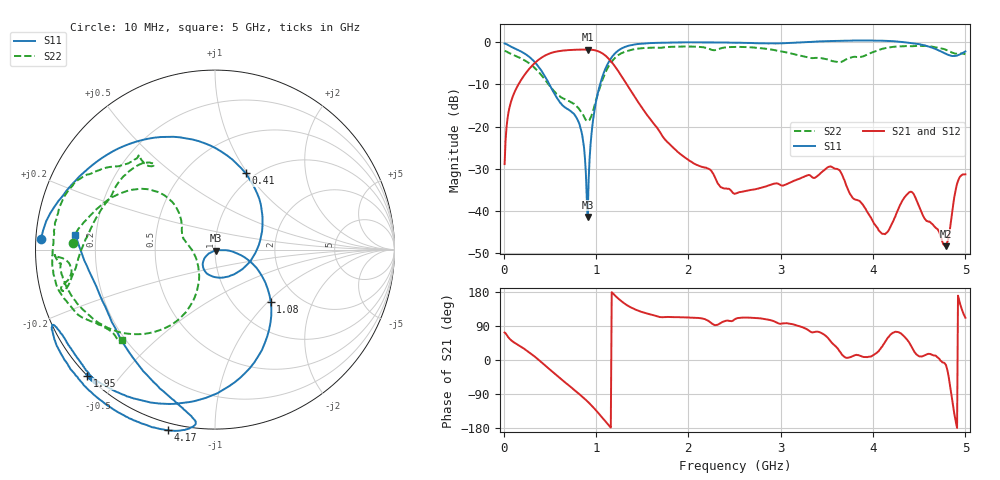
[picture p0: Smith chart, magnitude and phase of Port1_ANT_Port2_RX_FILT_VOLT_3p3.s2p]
! Created Tue Sep 16 09:50:58 2025
# hz S ma R 50
! 2 Port Network Data from SP1.SP block
! freq  magS11  angS11  magS21  angS21  magS12  angS12  magS22  angS22
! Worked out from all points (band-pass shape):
!   500 points, 10 MHz to 5 GHz, reference 50 ohm
!   highest |S21| = -1.70 dB at 910 MHz (marker M1); lowest = -48.5 dB at 4.79 GHz (marker M2)
!   |S21| within 3 dB of the highest: 346.7 MHz to 1.17 GHz (823 MHz wide, 109 % of centre)
!   lowest |S11| = -41.5 dB at 910 MHz (marker M3), VSWR 1.02, Z = 50.6 - j0.623 ohm
!   |S11| at or under -10 dB: 495.9 MHz to 1.043 GHz (547.5 MHz wide, 71.1 % of centre)
!   |S22| runs from -18.7 to -0.8 dB; largest |S21 - S12| = 0.0009
!   S11 on the Smith chart (normalised r, x): 10 MHz: 0.01, +0.03; 410 MHz: 0.91, +0.98; 1.08 GHz: 1.47, -1.04; 1.95 GHz: -0.00, -0.41; 4.17 GHz: -0.03, -0.77; 5 GHz: 0.12, +0.05
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1e7  0.9715 176.6  0.03572 72.5  0.03537 72.1  0.7932 177.4
5e7  0.9271 165.3  0.1432 59.9  0.1433 59.9  0.7571 169.9
1e8  0.8678 153.9  0.2304 48.4  0.2305 48.3  0.7117 163.5
2.7e8  0.6818 112.9  0.4755 21.4  0.4755 21.4  0.5709 144.3
4.1e8  0.4592 68.2  0.6589 -6.1  0.6591 -6.1  0.4058 132.8
6.3e8  0.1821 -40.5  0.7969 -52.2  0.7968 -52.2  0.2199 147.3
8.5e8  0.07959 -139.8  0.8221 -96.6  0.822 -96.6  0.1433 173.7
9.1e8  0.008432 -47.0  0.8225 -109.9  0.8227 -109.9  0.1158 -159.9
9.8e8  0.1465 -12.0  0.8099 -127.5  0.8101 -127.5  0.1703 -121.1
1.08e9  0.4245 -43.0  0.7266 -155.7  0.7268 -155.7  0.3861 -115.0
1.28e9  0.8512 -97.6  0.3916 154.3  0.3918 154.3  0.7479 -145.2
1.68e9  0.9879 -134.2  0.09015 114.2  0.09007 114.1  0.8631 -174.8
1.95e9  1.001 -135.3  0.04379 112.5  0.04402 112.5  0.8933 -177.8
2.51e9  0.9904 -132.4  0.01593 108.5  0.01592 108.5  0.8843 -165.9
2.92e9  0.9745 -147.9  0.02074 103.0  0.02081 102.6  0.8154 -168.9
3.34e9  1.016 -152.9  0.025 72.9  0.02499 72.8  0.6504 152.7
3.63e9  1.044 -138.5  0.03059 25.7  0.03067 25.7  0.5798 125.9
4.17e9  1.039 -104.7  0.005852 61.1  0.005813 61.9  0.869 155.6
4.41e9  0.9835 -96.5  0.01678 37.8  0.01675 37.8  0.902 176.3
4.79e9  0.7314 -134.2  0.003779 -13.4  0.003869 -15.0  0.8163 -151.7
4.91e9  0.6977 -165.6  0.02087 -179.5  0.02102 -179.3  0.7345 -139.3
5e9  0.7813 174.2  0.02699 111.5  0.02712 111.5  0.723 -136.0
